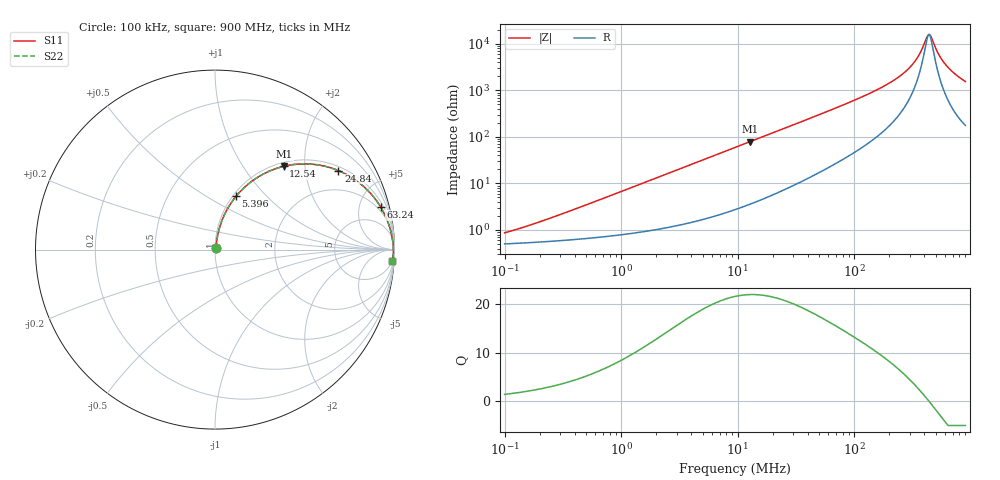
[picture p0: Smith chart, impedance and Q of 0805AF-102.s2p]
# MHz  S  MA  R  50
!Freq  MagS11  AngS11  MagS21  AngS21  MagS12  AngS12  MagS22  AngS22
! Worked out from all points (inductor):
!   801 points, 100 kHz to 900 MHz, reference 50 ohm
!   read as one part in series: L = 1.1 uH near 248.8 kHz
!   highest Q = 22 at 12.68 MHz (marker M1), where L = 985 nH
!   self-resonance near 433.8 MHz
!   S11 on the Smith chart (normalised r, x): 100 kHz: 1.01, +0.01; 5.396 MHz: 1.04, +0.68; 12.54 MHz: 1.07, +1.55; 24.84 MHz: 1.14, +3.02; 63.24 MHz: 1.47, +7.59; 900 MHz: 5, -31
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0.1  0.008653 54.3  0.995 -0.4  0.995 -0.4  0.008653 54.3
0.4603917  0.03179 76.6  0.9931 -1.8  0.9931 -1.8  0.03179 76.6
2.09559  0.1345 77.9  0.9808 -7.7  0.9808 -7.7  0.1345 77.9
5.39572  0.3194 68.5  0.9313 -18.6  0.9313 -18.6  0.3194 68.5
9.538608  0.5018 57.3  0.8421 -30.1  0.8421 -30.1  0.5018 57.3
12.53875  0.6005 50.5  0.7728 -36.9  0.7728 -36.9  0.6005 50.5
12.68244  0.6046 50.2  0.7696 -37.2  0.7696 -37.2  0.6046 50.2
24.84144  0.8161 32.7  0.5402 -54.6  0.5402 -54.6  0.8161 32.7
43.41739  0.9173 20.5  0.3512 -66.3  0.3512 -66.3  0.9173 20.5
63.237  0.9527 14.5  0.2506 -72.0  0.2506 -72.0  0.9527 14.5
123.8641  0.9813 7.2  0.1265 -77.9  0.1265 -77.9  0.9813 7.2
197.6253  0.9892 4.0  0.07029 -79.1  0.07029 -79.1  0.9892 4.0
259.7835  0.9916 2.5  0.04424 -77.9  0.04424 -77.9  0.9916 2.5
315.3114  0.9928 1.5  0.02773 -74.2  0.02773 -74.2  0.9928 1.5
357.4173  0.9933 0.9  0.01777 -67.4  0.01777 -67.4  0.9933 0.9
419.235  0.9937 0.2  0.007256 -29.5  0.007256 -29.5  0.9937 0.2
438.7856  0.9938 -0.0  0.006245 0.7  0.006245 0.7  0.9938 -0.0
459.248  0.9938 -0.2  0.007247 31.0  0.007247 31.0  0.9938 -0.2
526.5405  0.9938 -0.9  0.01611 66.8  0.01611 66.8  0.9938 -0.9
603.6933  0.9935 -1.5  0.02707 75.3  0.02707 75.3  0.9935 -1.5
724.4289  0.9926 -2.4  0.04294 78.9  0.04294 78.9  0.9926 -2.4
900  0.9907 -3.6  0.06387 79.8  0.06387 79.8  0.9907 -3.6
